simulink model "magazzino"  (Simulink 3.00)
settings: Solver=ode45  StartTime=0.0  StopTime=50  MaxStep=0.01  RelTol=1e-5  AbsTol=1e-5

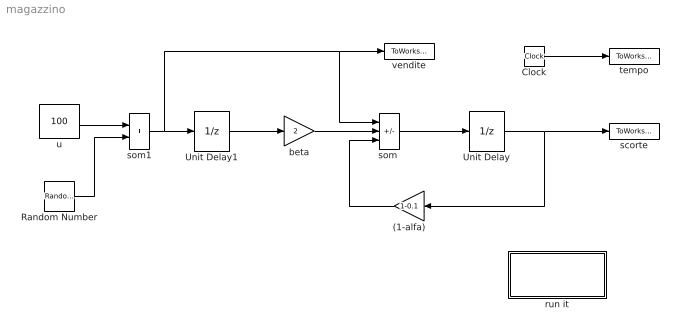
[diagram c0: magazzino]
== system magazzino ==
  (1-alfa) : Gain  Orientation=left  Gain=1-0.1  SaturateOnIntegerOverflow=on
  Clock : Clock
  Random Number : RandomNumber  Mean=0  Variance=1000  Seed=0  SampleTime=1
  Unit Delay : UnitDelay  X0=200  SampleTime=1
  Unit Delay1 : UnitDelay  X0=100  SampleTime=1
  beta : Gain  Gain=2  SaturateOnIntegerOverflow=on
  run it : Subsystem  Description=plot
  scorte : ToWorkspace  VariableName=s  SampleTime=1  SaveFormat=Matrix
  "som " : Sum  Inputs=-++  SaturateOnIntegerOverflow=on
  som1 : Sum  Inputs=++  SaturateOnIntegerOverflow=on
  tempo : ToWorkspace  VariableName=k  SampleTime=1  SaveFormat=Matrix
  u : Constant  Value=100
  vendite : ToWorkspace  VariableName=v  SampleTime=1  SaveFormat=Matrix
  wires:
  "som "/1 -> Unit Delay/1
  Clock/1 -> tempo/1
  Unit Delay/1 -> scorte/1, (1-alfa)/1
  (1-alfa)/1 -> "som "/3
  beta/1 -> "som "/2
  Unit Delay1/1 -> beta/1
  som1/1 -> Unit Delay1/1, vendite/1, "som "/1
  u/1 -> som1/1
  Random Number/1 -> som1/2

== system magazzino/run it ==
